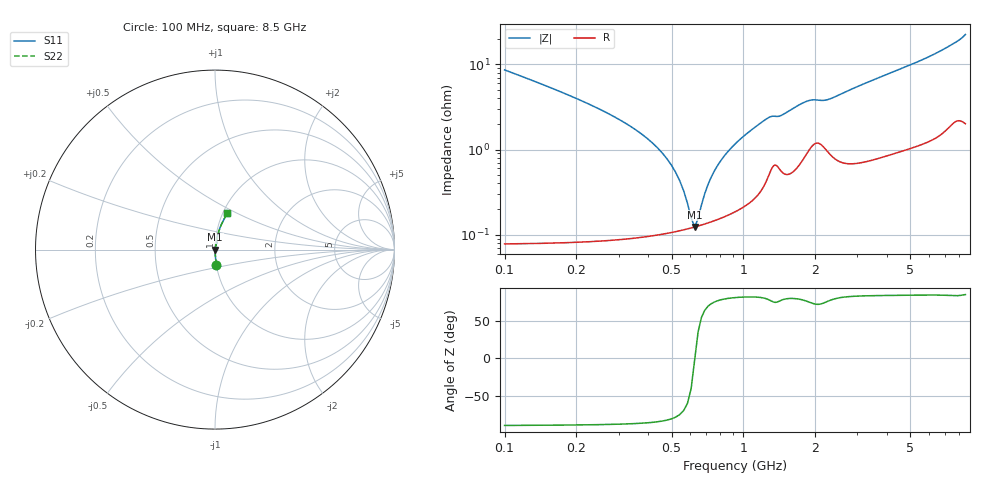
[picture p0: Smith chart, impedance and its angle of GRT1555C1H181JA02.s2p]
!Murata Part Number: GRT1555C1H181JA02
!These Parameters are Measured in Series Mode Connection
!Data Generated on Jun 19, 2026
!  o--ll--o
!Port1  Port2
!  o------o
!Operation Temp=25[degC], DC Bias Voltage=0[V]
!Freq. Start=100[MHz] Stop=9[GHz] 401[Steps]
# Hz S RI R 50
!Freq.(Hz) S11(Real) S11(Imag) S21(Real) S21(Imag) S12(Real) S12(Imag) S22(Real) S22(Imag)
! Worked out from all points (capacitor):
!   401 points, 100 MHz to 8.5 GHz, reference 50 ohm
!   read as one part in series: C = 180 pF near 142 MHz
!   lowest |Z| = 123 mohm at 625 MHz (marker M1)
!   series resonance near 626.1 MHz, so ESL is about 360 pH
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1e8  0.00813 -0.0854  0.9919 0.0854  0.9919 0.0854  0.00813 -0.0854
4.57e8  0.00109 -0.00905  0.9989 0.00905  0.9989 0.00905  0.00109 -0.00905
5.2e8  0.00111 -0.00529  0.9989 0.00529  0.9989 0.00529  0.00111 -0.00529
5.83e8  0.00117 -0.00202  0.9988 0.00202  0.9988 0.00202  0.00117 -0.00202
6.04e8  0.0012 -0.00102  0.9988 0.00102  0.9988 0.00102  0.0012 -0.00102
6.25e8  0.00123 -4.88e-05  0.9988 4.88e-05  0.9988 4.88e-05  0.00123 -4.88e-05
6.46e8  0.00126 0.000889  0.9987 -0.000889  0.9987 -0.000889  0.00126 0.000889
6.67e8  0.0013 0.0018  0.9987 -0.0018  0.9987 -0.0018  0.0013 0.0018
7.09e8  0.00138 0.00355  0.9986 -0.00355  0.9986 -0.00355  0.00138 0.00355
7.72e8  0.00152 0.00602  0.9985 -0.00602  0.9985 -0.00602  0.00152 0.00602
8.35e8  0.00169 0.00835  0.9983 -0.00835  0.9983 -0.00835  0.00169 0.00835
9.19e8  0.00197 0.0113  0.998 -0.0113  0.998 -0.0113  0.00197 0.0113
1.045e9  0.00252 0.0156  0.9975 -0.0156  0.9975 -0.0156  0.00252 0.0156
1.234e9  0.00446 0.0219  0.9955 -0.0219  0.9955 -0.0219  0.00446 0.0219
1.507e9  0.00576 0.0263  0.9942 -0.0263  0.9942 -0.0263  0.00576 0.0263
1.864e9  0.0106 0.0354  0.9894 -0.0354  0.9894 -0.0354  0.0106 0.0354
2.242e9  0.0108 0.0365  0.9892 -0.0365  0.9892 -0.0365  0.0108 0.0365
2.914e9  0.00947 0.0517  0.9905 -0.0517  0.9905 -0.0517  0.00947 0.0517
4.3e9  0.0155 0.0805  0.9845 -0.0805  0.9845 -0.0805  0.0155 0.0805
5.707e9  0.0243 0.1112  0.9757 -0.1112  0.9757 -0.1112  0.0243 0.1112
7.114e9  0.04 0.1488  0.96 -0.1488  0.96 -0.1488  0.04 0.1488
8.5e9  0.0647 0.2052  0.9353 -0.2052  0.9353 -0.2052  0.0647 0.2052
